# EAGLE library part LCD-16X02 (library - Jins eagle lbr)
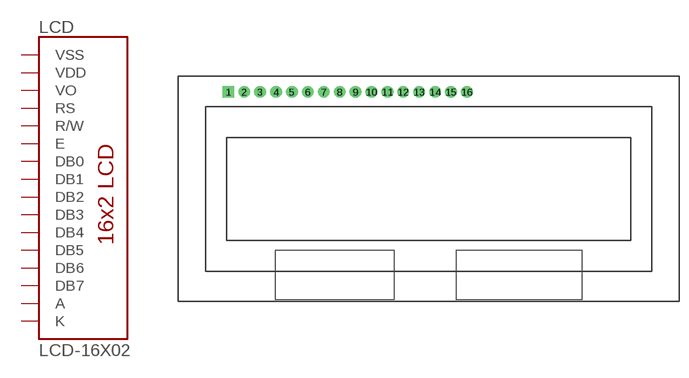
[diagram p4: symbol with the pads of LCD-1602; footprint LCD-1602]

Designator prefix LCD

## LCD-16X02LCD  [LCD-1602]
1  VSS  pwr
2  VDD  pwr
3  VO
4  RS  in
5  R/W  in
6  E  in
7  DB0
8  DB1
9  DB2
10  DB3
11  DB4
12  DB5
13  DB6
14  DB7
15  A  pwr
16  K  pwr

## Footprint LCD-1602 (pad centres in mm)
drill 1.016 pad 1.88 square: 1 -29.46,14.23
drill 1.016 pad 1.88: 2 -26.92,14.23; 3 -24.38,14.23; 4 -21.84,14.23; 5 -19.3,14.23; 6 -16.76,14.23; 7 -14.22,14.23; 8 -11.68,14.23; 9 -9.14,14.23; 10 -6.6,14.23; 11 -4.06,14.23; 12 -1.52,14.23; 13 1.02,14.23; 14 3.56,14.23; 15 6.1,14.23; 16 8.64,14.23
